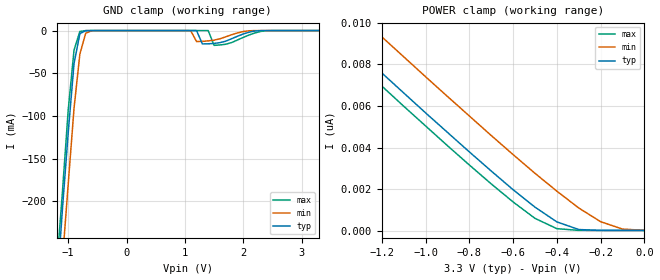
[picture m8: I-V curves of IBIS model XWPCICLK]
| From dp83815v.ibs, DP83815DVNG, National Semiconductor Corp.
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|   Model XWPCICLK
[Model]   XWPCICLK
Model_type   Input
Vinl =   0.80V
Vinh =   2.00V
Vmeas =   1.50V
Cref =  10.00pF
Rref =  50.00
C_comp   5.83pF   5.83pF   5.83pF
[Temperature Range]   27.00   100.00   0.000
[Voltage Range]   3.30V   3.00V   3.60V
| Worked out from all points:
|   GND clamp passes 1 mA (typ) near -0.73 V on its own axis
[GND_clamp]
| voltage   I(typ)   I(min)   I(max)
-3.3V     -2.58A     -2.63A     -2.56A
-1.2V     -310mA     -370mA     -280mA
-1.1V     -210mA     -270mA     -190mA
-1V       -120mA     -180mA     -93.33mA
-900mV    -38.51mA   -90.99mA   -22.84mA
-800mV    -3.61mA    -27.5mA    -1.07mA
-600mV    -3.26uA    -200uA     -430nA
1.1V      -32.95nA   -170uA     -13.32pA
1.2V      -2.54uA    -12.84mA   -180pA
1.4V      -15.49mA   -12.08mA   -21.11uA
1.5V      -15.01mA   -11.19mA   -17.3mA
3.3V      6.6pA      1.09nA     6pA
[POWER_clamp]
| voltage   I(typ)   I(min)   I(max)
-3.3V     28.22nA    29.93nA    27.61nA
-1.5V     10.5nA     12.24nA    9.87nA
-1.4V     9.53nA     11.27nA    8.89nA
-1.3V     8.56nA     10.3nA     7.92nA
-1.2V     7.59nA     9.33nA     6.96nA
-800mV    3.79nA     5.52nA     3.16nA
-500mV    1.13nA     2.76nA     590pA
-400mV    420pA      1.9nA      93.79pA
-300mV    51.69pA    1.09nA     10.86pA
-200mV    8.93pA     430pA      8.09pA
-100mV    7.08pA     73.99pA    7.65pA
0V        6.6pA      11.6pA     7.2pA
